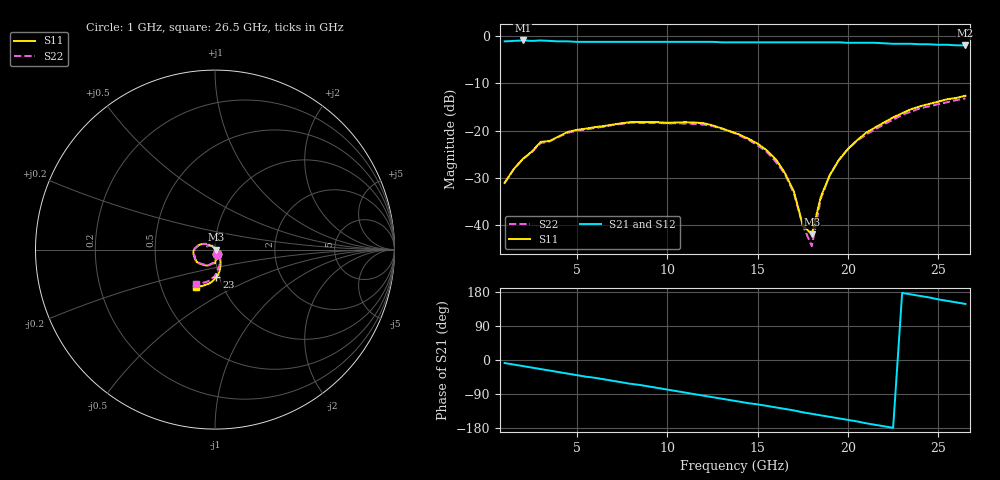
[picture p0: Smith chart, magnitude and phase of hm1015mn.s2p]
! HMMC-1015
! S-PARAMETERS at  Minimum Attenuation;  V1 =  0V;  V2 = -4V.  LAST  UPDATED  02-25-97
#  GHZ  S  MA  R  50
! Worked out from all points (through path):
!   52 points, 1 GHz to 26.5 GHz, reference 50 ohm
!   highest |S21| = -0.92 dB at 2 GHz (marker M1); lowest = -1.9 dB at 26.5 GHz (marker M2)
!   group delay of S21, straight-line fit = 22.1 ps
!   lowest |S11| = -41.9 dB at 18 GHz (marker M3), VSWR 1.02, Z = 50.8 + j0.0142 ohm
!   |S11| at or under -10 dB: start of sweep to end of sweep
!   |S22| runs from -44.4 to -13.2 dB; largest |S21 - S12| = 0.016
!   S11 on the Smith chart (normalised r, x): 1 GHz: 1.02, -0.05; 23 GHz: 0.97, -0.30; 26.5 GHz: 0.75, -0.33
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1  0.028 -71.0  0.88 -8.0  0.88 -8.0  0.028 -71.0
2  0.05 -72.0  0.9 -16.0  0.9 -16.0  0.05 -71.0
3  0.076 -90.0  0.9 -24.0  0.9 -25.0  0.074 -90.0
5.5  0.105 -125.0  0.87 -44.0  0.87 -44.0  0.103 -126.0
8  0.123 -147.0  0.87 -63.0  0.87 -63.0  0.122 -148.0
9.5  0.123 -158.0  0.87 -74.0  0.87 -74.0  0.121 -159.0
12  0.12 -177.0  0.87 -94.0  0.87 -94.0  0.116 -177.0
14  0.091 163.0  0.86 -110.0  0.86 -110.0  0.089 163.0
15.5  0.062 150.0  0.86 -121.0  0.86 -121.0  0.06 147.0
16.5  0.036 138.0  0.86 -129.0  0.86 -129.0  0.035 134.0
17  0.023 130.0  0.86 -133.0  0.86 -133.0  0.022 124.0
17.5  0.01 105.0  0.86 -138.0  0.86 -138.0  0.01 108.0
18  0.008 1.0  0.86 -142.0  0.86 -142.0  0.006 -19.0
18.5  0.02 -37.0  0.86 -146.0  0.86 -146.0  0.019 -48.0
19  0.034 -49.0  0.86 -150.0  0.86 -150.0  0.034 -54.0
19.5  0.049 -56.0  0.86 -154.0  0.86 -154.0  0.049 -58.0
20  0.064 -62.0  0.85 -158.0  0.85 -158.0  0.064 -64.0
21  0.095 -71.0  0.85 -167.0  0.85 -166.0  0.091 -74.0
22.5  0.138 -82.0  0.83 -179.0  0.84 -179.0  0.131 -87.0
23  0.153 -87.0  0.83 177.0  0.83 177.0  0.147 -90.0
24.5  0.192 -100.0  0.82 165.0  0.82 165.0  0.181 -103.0
26.5  0.234 -117.0  0.8 148.0  0.8 149.0  0.219 -119.0
